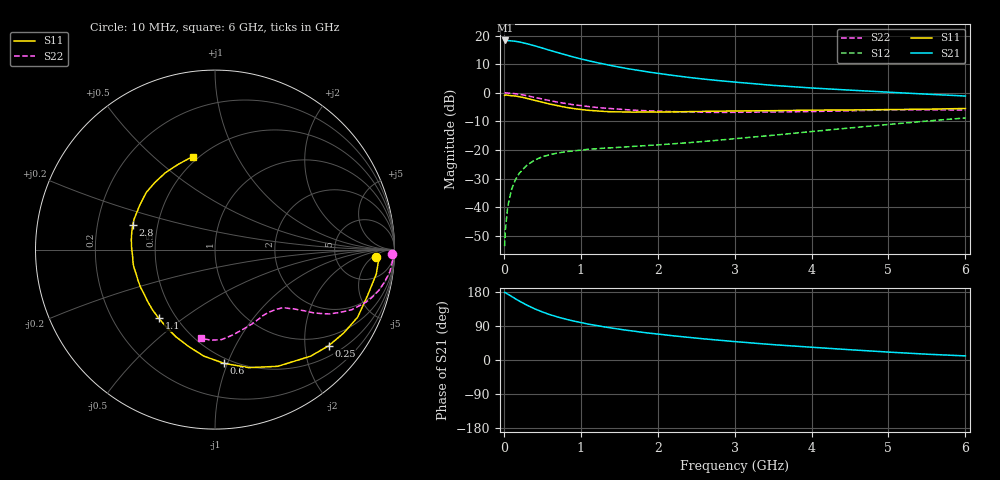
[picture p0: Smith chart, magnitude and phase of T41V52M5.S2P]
! Infineon Technologies  Discrete & RF Semiconductors
! BFR182T
! Si NPN RF Bipolar Junction Transistor in SC75
! VCE = 1.5 V  IC = 2.5 mA
! Common Emitter S-Parameters:  October  1999
# GHz  S  MA  R  50
!  f  S11  S21  S12  S22
! GHz  MAG  ANG  MAG  ANG  MAG  ANG  MAG  ANG
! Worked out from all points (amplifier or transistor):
!   36 points, 10 MHz to 6 GHz, reference 50 ohm
!   highest |S21| = 18.3 dB at 20 MHz (marker M1)
!   |S21| within 3 dB of that: start of sweep to 543.1 MHz
!   unconditionally stable (mu >= 1): 1.795 GHz to 4.349 GHz
!   at 250 MHz: K = 0.17, MSG = 22.1 dB, |S12| = -26.7 dB
!   at 1.4 GHz: K = 0.86, MSG = 14.3 dB, |S12| = -19.2 dB
!   at 6 GHz: K = 0.85, MSG = 3.8 dB, |S12| = -8.8 dB
!   lowest NFmin = 1.10 dB at 450 MHz
!   S11 on the Smith chart (normalised r, x): 10 MHz: 15, -7; 250 MHz: 0.74, -2.54; 600 MHz: 0.46, -0.97; 1.1 GHz: 0.40, -0.41; 2.8 GHz: 0.36, +0.13; 6 GHz: 0.47, +0.67
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0.01  0.8983 -2.8  8.154 178.2  0.0021 80.6  0.9886 -1.5
0.02  0.9162 -2.2  8.208 177.8  0.004 94.8  0.9999 -1.5
0.05  0.909 -8.6  8.178 173.8  0.0102 88.0  0.9911 -3.7
0.1  0.8881 -16.5  8.062 167.9  0.0205 80.9  0.9821 -7.2
0.2  0.8547 -32.9  7.742 155.7  0.0392 73.0  0.9431 -13.7
0.25  0.8292 -40.3  7.472 150.2  0.0465 68.4  0.9166 -16.7
0.3  0.7977 -48.1  7.204 144.8  0.0543 65.6  0.8907 -19.2
0.4  0.7384 -61.7  6.629 135.1  0.0668 58.8  0.8329 -23.7
0.5  0.6843 -74.0  6.049 126.9  0.0765 54.2  0.779 -26.7
0.6  0.6352 -85.6  5.511 119.6  0.0833 50.4  0.7302 -29.4
0.7  0.5966 -96.0  5.036 113.5  0.0889 47.6  0.6874 -31.2
0.8  0.5596 -105.2  4.62 108.0  0.0933 45.7  0.6521 -32.7
0.9  0.5325 -114.1  4.238 103.2  0.0967 44.3  0.6204 -33.8
1.1  0.4944 -129.3  3.642 94.6  0.1036 42.7  0.5758 -35.7
1.3  0.4736 -142.5  3.185 87.6  0.1081 42.2  0.5411 -37.4
1.6  0.4616 -158.7  2.656 78.4  0.1138 42.8  0.5067 -39.8
2.2  0.4644 179.1  2.012 63.9  0.1289 47.4  0.4703 -46.0
2.8  0.4782 163.5  1.631 52.2  0.1491 51.9  0.4543 -53.8
3.5  0.4874 149.0  1.349 40.5  0.1814 55.9  0.4626 -63.3
4.5  0.502 132.0  1.114 27.1  0.2437 57.0  0.4858 -78.3
5.5  0.5179 113.0  0.947 15.3  0.3215 54.0  0.5052 -92.5
6  0.5327 103.6  0.879 10.8  0.3639 50.8  0.5004 -98.9
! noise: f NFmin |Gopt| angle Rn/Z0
0.45  1.1  0.39  29  0.35
0.9  1.2  0.37  59  0.28
1.8  1.8  0.28  128  0.2
